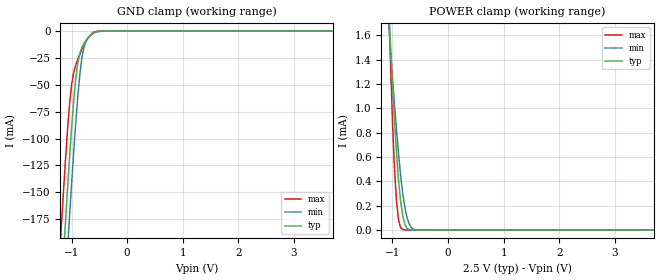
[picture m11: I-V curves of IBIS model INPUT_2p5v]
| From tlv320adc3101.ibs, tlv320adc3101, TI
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|   INPUT_2p5v
[Model]   INPUT_2p5v
Model_type   Input
Vinl = 0.75
Vinh = 1.75
|   typ   min   max
C_comp   1.022pF   1.010pF   1.056pF
[Voltage Range]   2.5   2.25   2.75
[Temperature Range]   27   85   -40
[Power Clamp Reference]   2.5   2.25   2.75
[GND Clamp Reference]   -0   -0   -0
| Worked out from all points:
|   GND clamp passes 1 mA (typ) near -0.57 V on its own axis
|   POWER clamp passes 1 mA (typ) near -0.97 V on its own axis
[GND Clamp]
|   Voltage   I(typ)   I(min)   I(max)
-2.5V     -1.509A    -1.565A    -1.451A
-1.188V   -246.6mA   -304.5mA   -185.3mA
-1.113V   -180.8mA   -237.6mA   -122.2mA
-1.075V   -149.1mA   -205mA     -93.63mA
-1.038V   -118.9mA   -173.2mA   -68.82mA
-1V       -90.51mA   -142.3mA   -50.08mA
-925mV    -44.19mA   -85.31mA   -31.51mA
-887.5mV  -29.35mA   -60.54mA   -26.15mA
-812.5mV  -15.2mA    -24.36mA   -16.89mA
-775mV    -11.52mA   -14.62mA   -12.78mA
-587.5mV  -1.243mA   -1.427mA   -757.6uA
4.963V    0A         0A         0A
[POWER Clamp]
|   Voltage   I(typ)   I(min)   I(max)
-2.5V     16.68mA    11.85mA    28.34mA
-1.075V   1.887mA    1.735mA    1.989mA
-1.038V   1.542mA    1.493mA    1.414mA
-1V       1.21mA     1.257mA    900.7uA
-962.5mV  899.7uA    1.029mA    493.8uA
-925mV    621.7uA    812.9uA    225.3uA
-887.5mV  393.1uA    612.6uA    75.87uA
-812.5mV  111.7uA    291.4uA    3.309uA
-775mV    44.39uA    181.7uA    584nA
-700mV    3.907uA    49.68uA    8.869nA
-587.5mV  60.81nA    2.448uA    0A
4.963V    0A         0A         0A
